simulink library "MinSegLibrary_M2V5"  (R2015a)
settings: Solver=ode45  StartTime=0.0  StopTime=10.0  RelTol=1e-3
undefined symbols (not defined in the file or in its folder): PWMoffset, Vsupply
libraries: arduinolib x8

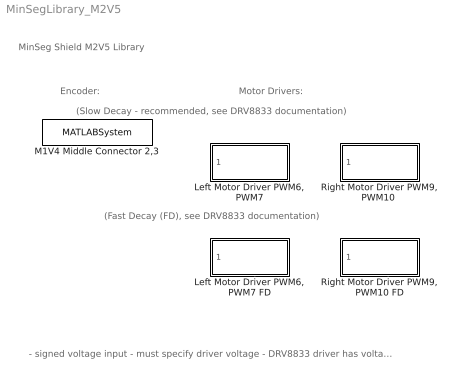
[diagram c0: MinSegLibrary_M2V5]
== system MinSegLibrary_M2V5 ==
  note: Encoder:
  note: MinSeg Shield M2V5 Library
  note: (Slow Decay - recommended, see DRV8833 documentation)
  note: Motor Drivers:
  note: (Fast Decay (FD), see DRV8833 documentation)
  note: - signed voltage input - must specify driver voltage - DRV8833 driver has voltage drop of about 0.6 volts, so max usable USB voltage is about 3.9 volts - Fast decay is nonlinear PWM to voltage for NXT motor - look at generic driver block in RASPlib for table lookup and other options
  "Left Motor Driver PWM6, PWM7" : Subsystem
  "Left Motor Driver PWM6, PWM7 FD" : Subsystem
  M1V4 Middle Connector 2,3 : MATLABSystem  System=Encoder_arduino  Encoder=0  PinA=3  PinB=2
  "Right Motor Driver PWM9, PWM10 " : Subsystem
  "Right Motor Driver PWM9, PWM10 FD" : Subsystem

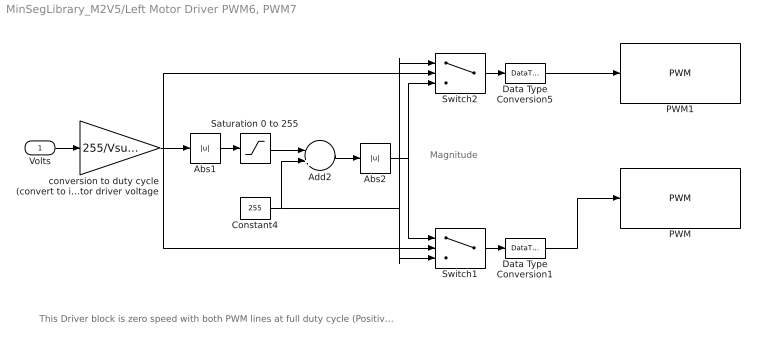
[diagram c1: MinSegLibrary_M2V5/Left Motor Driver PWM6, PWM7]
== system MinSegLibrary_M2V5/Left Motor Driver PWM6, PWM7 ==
  note: This Driver block is zero speed with both PWM lines at full duty cycle (Positive voltage on both motor terminals). This method produces a linear motor response for DRV8833 driver in both directions and eliminates the typical dead zone when the motor starts. The driver may draw more current in this configuration (has not been verified) The SN754410 driver this has no effect, so the driver could alternatively be modified so that zero speed is zero voltage to both PWM lines.
  note: Magnitude
  Volts : Inport
  Abs1 : Abs
  Abs2 : Abs
  Add2 : Sum  Inputs=-+
  Constant4 : Constant  Value=255
  Data Type Conversion1 : DataTypeConversion  OutDataTypeStr=uint8
  Data Type Conversion5 : DataTypeConversion  OutDataTypeStr=uint8
  PWM : arduinolib/PWM  pinNumber=7  blockPlatform=arduino
  PWM1 : arduinolib/PWM  pinNumber=6  blockPlatform=arduino
  Saturation 0 to 255 : Saturate  UpperLimit=255  LowerLimit=0
  Switch1 : Switch
  Switch2 : Switch
  conversion to duty cycle (convert to int) denominator is motor driver voltage : Gain  Gain=255/Vsupply  OutDataTypeStr=int16
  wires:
  Volts/1 -> conversion to duty cycle (convert to int) denominator is motor driver voltage/1
  conversion to duty cycle (convert to int) denominator is motor driver voltage/1 -> Switch2/2, Abs1/1, Switch1/2
  Saturation 0 to 255/1 -> Add2/1
  Abs1/1 -> Saturation 0 to 255/1
  Constant4/1 -> Switch1/3, Switch2/1, Add2/2
  Add2/1 -> Abs2/1
  Abs2/1 -> Switch2/3, Switch1/1
  Switch2/1 -> Data Type Conversion5/1
  Switch1/1 -> Data Type Conversion1/1
  Data Type Conversion5/1 -> PWM1/1
  Data Type Conversion1/1 -> PWM/1

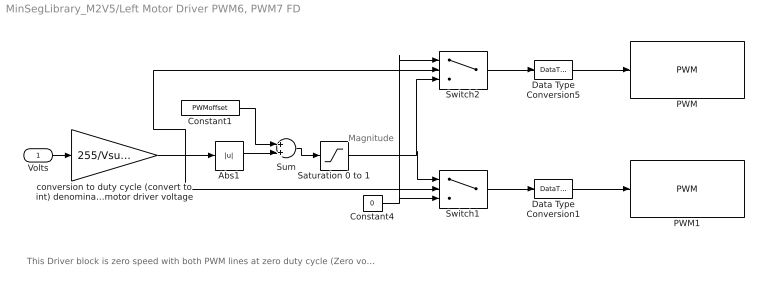
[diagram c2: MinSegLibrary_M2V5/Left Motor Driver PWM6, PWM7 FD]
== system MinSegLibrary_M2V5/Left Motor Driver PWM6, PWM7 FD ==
  note: This Driver block is zero speed with both PWM lines at zero duty cycle (Zero voltage on both motor terminals). This method produces a nonlinear motor response for DRV8833 driver in both directions and eliminates
  note: Magnitude
  Volts : Inport
  Abs1 : Abs
  Constant1 : Constant  Value=PWMoffset
  Constant4 : Constant  Value=0
  Data Type Conversion1 : DataTypeConversion  OutDataTypeStr=uint8
  Data Type Conversion5 : DataTypeConversion  OutDataTypeStr=uint8
  PWM : arduinolib/PWM  pinNumber=6  blockPlatform=arduino
  PWM1 : arduinolib/PWM  pinNumber=7  blockPlatform=arduino
  Saturation 0 to 1 : Saturate  UpperLimit=255  LowerLimit=0
  Sum : Sum
  Switch1 : Switch
  Switch2 : Switch
  conversion to duty cycle (convert to int) denominator is motor driver voltage : Gain  Gain=255/Vsupply  OutDataTypeStr=int16
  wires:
  Volts/1 -> conversion to duty cycle (convert to int) denominator is motor driver voltage/1
  conversion to duty cycle (convert to int) denominator is motor driver voltage/1 -> Switch1/2, Abs1/1, Switch2/2
  Constant4/1 -> Switch2/1, Switch1/3
  Saturation 0 to 1/1 -> Switch2/3, Switch1/1
  Switch2/1 -> Data Type Conversion5/1
  Switch1/1 -> Data Type Conversion1/1
  Data Type Conversion5/1 -> PWM/1
  Data Type Conversion1/1 -> PWM1/1
  Abs1/1 -> Sum/2
  Sum/1 -> Saturation 0 to 1/1
  Constant1/1 -> Sum/1

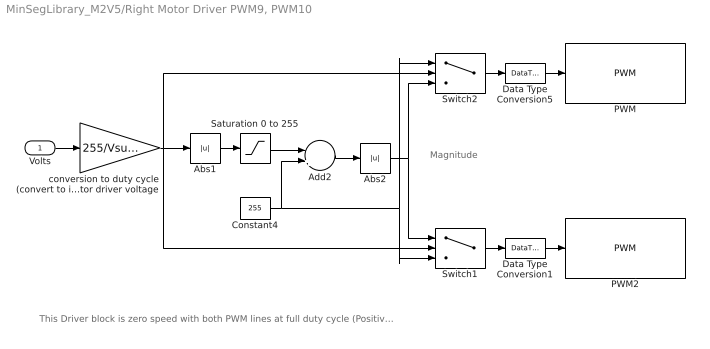
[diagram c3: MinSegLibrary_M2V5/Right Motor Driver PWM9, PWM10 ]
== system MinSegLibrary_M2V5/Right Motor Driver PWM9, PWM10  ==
  note: This Driver block is zero speed with both PWM lines at full duty cycle (Positive voltage on both motor terminals). This method produces a linear motor response for DRV8833 driver in both directions and eliminates the typical dead zone when the motor starts. The driver may draw more current in this configuration (has not been verified) The SN754410 driver this has no effect, so the driver could alternatively be modified so that zero speed is zero voltage to both PWM lines.
  note: Magnitude
  Volts : Inport
  Abs1 : Abs
  Abs2 : Abs
  Add2 : Sum  Inputs=-+
  Constant4 : Constant  Value=255
  Data Type Conversion1 : DataTypeConversion  OutDataTypeStr=uint8
  Data Type Conversion5 : DataTypeConversion  OutDataTypeStr=uint8
  PWM : arduinolib/PWM  pinNumber=9  blockPlatform=arduino
  PWM2 : arduinolib/PWM  pinNumber=10  blockPlatform=arduino
  Saturation 0 to 255 : Saturate  UpperLimit=255  LowerLimit=0
  Switch1 : Switch
  Switch2 : Switch
  conversion to duty cycle (convert to int) denominator is motor driver voltage : Gain  Gain=255/Vsupply  OutDataTypeStr=int16
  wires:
  Volts/1 -> conversion to duty cycle (convert to int) denominator is motor driver voltage/1
  conversion to duty cycle (convert to int) denominator is motor driver voltage/1 -> Abs1/1, Switch2/2, Switch1/2
  Saturation 0 to 255/1 -> Add2/1
  Abs1/1 -> Saturation 0 to 255/1
  Constant4/1 -> Switch1/3, Switch2/1, Add2/2
  Add2/1 -> Abs2/1
  Abs2/1 -> Switch2/3, Switch1/1
  Switch2/1 -> Data Type Conversion5/1
  Switch1/1 -> Data Type Conversion1/1
  Data Type Conversion5/1 -> PWM/1
  Data Type Conversion1/1 -> PWM2/1

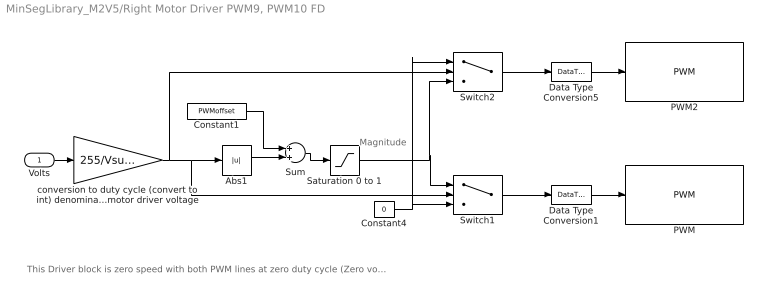
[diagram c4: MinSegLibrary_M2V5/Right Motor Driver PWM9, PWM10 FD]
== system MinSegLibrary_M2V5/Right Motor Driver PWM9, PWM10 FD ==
  note: This Driver block is zero speed with both PWM lines at zero duty cycle (Zero voltage on both motor terminals). This method produces a nonlinear motor response for DRV8833 driver in both directions and eliminates
  note: Magnitude
  Volts : Inport
  Abs1 : Abs
  Constant1 : Constant  Value=PWMoffset
  Constant4 : Constant  Value=0
  Data Type Conversion1 : DataTypeConversion  OutDataTypeStr=uint8
  Data Type Conversion5 : DataTypeConversion  OutDataTypeStr=uint8
  PWM : arduinolib/PWM  pinNumber=10  blockPlatform=arduino
  PWM2 : arduinolib/PWM  pinNumber=9  blockPlatform=arduino
  Saturation 0 to 1 : Saturate  UpperLimit=255  LowerLimit=0
  Sum : Sum
  Switch1 : Switch
  Switch2 : Switch
  conversion to duty cycle (convert to int) denominator is motor driver voltage : Gain  Gain=255/Vsupply  OutDataTypeStr=int16
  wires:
  Volts/1 -> conversion to duty cycle (convert to int) denominator is motor driver voltage/1
  conversion to duty cycle (convert to int) denominator is motor driver voltage/1 -> Switch1/2, Abs1/1, Switch2/2
  Constant4/1 -> Switch2/1, Switch1/3
  Saturation 0 to 1/1 -> Switch2/3, Switch1/1
  Switch2/1 -> Data Type Conversion5/1
  Switch1/1 -> Data Type Conversion1/1
  Data Type Conversion5/1 -> PWM2/1
  Data Type Conversion1/1 -> PWM/1
  Abs1/1 -> Sum/2
  Sum/1 -> Saturation 0 to 1/1
  Constant1/1 -> Sum/1
